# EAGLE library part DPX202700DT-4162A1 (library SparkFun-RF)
TDK - DPX202700DT-4162A1 Multilayer Diplexer For 698-960MHz / 1710-2700MHz 2.0x1.25mm [EIA 0805] Datasheet SparkFun Products LoRa Thing Plus - expLoRaBLE (WRL-17506) *Note, this uses the "standard" footprint (not the "-L" or "-M")
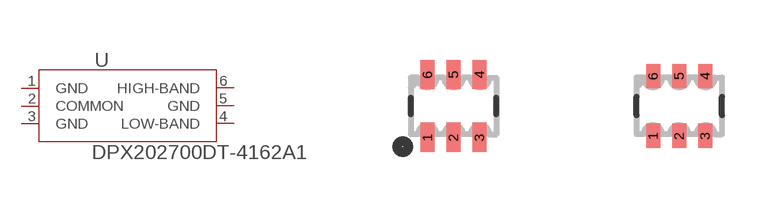
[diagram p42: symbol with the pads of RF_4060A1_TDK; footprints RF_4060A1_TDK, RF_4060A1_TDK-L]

Designator prefix U

## DPX202700DT-4162A1 (BUILT_BY: EMA_Matt; COPYRIGHT: Copyright (C) 2018 Accelerated Designs. All rights reserved; MANUFACTURER_PART_NUMBER: DPX202700DT-4162A1; PROD_ID: IC-15465; SOURCELIBRARY: TDK_2019-10-09; VENDOR: TDK)  [RF_4060A1_TDK]
1  GND  pas
2  COMMON  pas
3  GND  pas
4  LOW-BAND  pas
5  GND  pas
6  HIGH-BAND  pas

## DPX202700DT-4162A1RF_4060A1_TDK-L (BUILT_BY: EMA_Matt; COPYRIGHT: Copyright (C) 2018 Accelerated Designs. All rights reserved; MANUFACTURER_PART_NUMBER: DPX202700DT-4162A1; SOURCELIBRARY: TDK_2019-10-09; VENDOR: TDK)  [RF_4060A1_TDK-L]
Pads as for RF_4060A1_TDK

## DPX202700DT-4162A1RF_4060A1_TDK-M (BUILT_BY: EMA_Matt; COPYRIGHT: Copyright (C) 2018 Accelerated Designs. All rights reserved; MANUFACTURER_PART_NUMBER: DPX202700DT-4162A1; SOURCELIBRARY: TDK_2019-10-09; VENDOR: TDK)  [RF_4060A1_TDK-M]
Pads as for RF_4060A1_TDK

## Footprint RF_4060A1_TDK (pad centres in mm)
smd 0.356 x 0.737: 1 -0.65,-0.787; 2 0,-0.787; 3 0.65,-0.787; 4 0.65,0.787; 5 0,0.787; 6 -0.65,0.787

## Footprint RF_4060A1_TDK-L (pad centres in mm)
smd 0.356 x 0.61: 1 -0.65,-0.749; 2 0,-0.749; 3 0.65,-0.749; 4 0.65,0.749; 5 0,0.749; 6 -0.65,0.749

## Footprint RF_4060A1_TDK-M (pad centres in mm)
smd 0.406 x 0.864: 1 -0.65,-0.826; 2 0,-0.826; 3 0.65,-0.826; 4 0.65,0.826; 5 0,0.826; 6 -0.65,0.826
